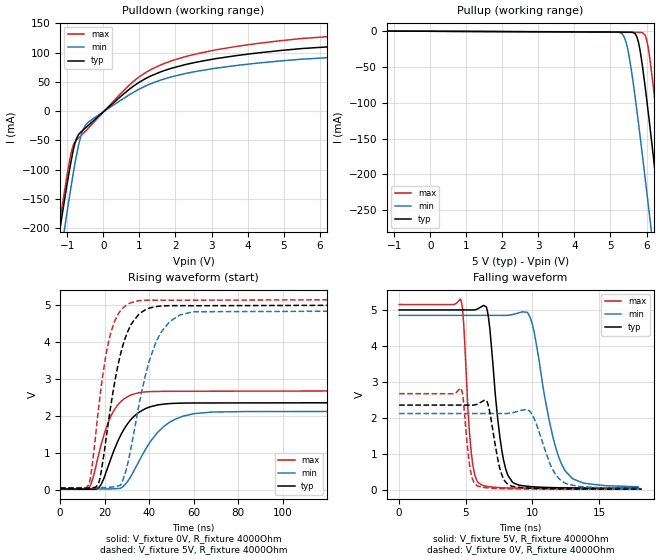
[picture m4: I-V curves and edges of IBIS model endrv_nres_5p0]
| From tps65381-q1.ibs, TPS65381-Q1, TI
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|   endrv_nres_5p0 Model
[Model]   endrv_nres_5p0
Model_type   Output
Polarity   Non-Inverting
Vmeas = 1.65
Vref = 2.5
Cref = 2pF
Rref = 50
|   typ   min   max
|   (nom PVT)   (fast PVT)   (slow PVT)
C_comp   1.702e-12   1.384e-12   1.872e-12
| Where nom  PVT is Nominal Process, 5V, 27C
|   Fast PVT is Strong Process,  5.15V, -40C
|   Slow PVT is Weak Process,   4.85V, 150C
[Voltage Range]   5   4.85   5.15
|Junction Temperature
[Temperature Range]   27   150   -40
[Pullup Reference]   5   4.85   5.15
[Pulldown Reference]   0   0   0
[Power Clamp Reference]   5   4.85   5.15
[GND Clamp Reference]   0   0   0
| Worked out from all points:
|   slope of the pulldown table from 0 to 0.75 V, typ, clamps not added: 18.8 ohm
|   slope of the pullup table from 0 to 0.75 V, typ, clamps not added: 4.48 kohm
|   falling waveform, V_fixture 5V, R_fixture 4000Ohm: 20-80 % time 815ps typ, 1.5ns min, 492ps max; typ from 5 V to 0.053 V
|   rising waveform, V_fixture 0V, R_fixture 4000Ohm: 20-80 % time 11ns typ, 14ns min, 8.45ns max; typ from 0.02 V to 2.36 V
|   rising waveform, V_fixture 5V, R_fixture 4000Ohm: 20-80 % time 8.92ns typ, 11ns min, 7.09ns max; typ from 0.043 V to 5 V
|   falling waveform, V_fixture 0V, R_fixture 4000Ohm: 20-80 % time 714ps typ, 1.29ns min, 445ps max; typ from 2.36 V to 0.025 V
[Pulldown]
|   Voltage   I(typ)   I(min)   I(max)
-5V       -1.931A    -1.927A    -1.96A
-1.232V   -211.8mA   -265.5mA   -197mA
-1.06V    -144.2mA   -193.9mA   -129.2mA
-882.3mV  -80.85mA   -123.2mA   -67.84mA
-760mV    -48.91mA   -79.67mA   -50.34mA
-625.3mV  -35.56mA   -42.43mA   -42.13mA
-500mV    -28.71mA   -24.43mA   -34.3mA
809.2mV   41.63mA    31.33mA    49.58mA
1.698V    69.52mA    55.27mA    81.68mA
2.617V    84.16mA    68.42mA    98.35mA
4.291V    99.53mA    82.16mA    115.8mA
10V       124.5mA    104.8mA    143.4mA
[Pullup]
|   Voltage   I(typ)   I(min)   I(max)
-5V       1.116mA    973.5uA    1.352mA
5.263V    -1.174mA   -1.864mA   -1.423mA
5.389V    -1.203mA   -9.349mA   -1.457mA
5.506V    -1.236mA   -32.1mA    -1.489mA
5.73V     -7.607mA   -109.9mA   -1.552mA
5.89V     -50.12mA   -175.1mA   -2.045mA
6.006V    -95.75mA   -224mA     -12.31mA
6.098V    -135.2mA   -263.8mA   -40.86mA
6.38V     -260.6mA   -385.9mA   -163.4mA
6.546V    -335.9mA   -458.5mA   -240.9mA
7.36V     -705.8mA   -815.7mA   -623.3mA
10V       -1.928A    -1.994A    -1.885A
[Ramp]
R_load = 4000
|   typ   min   max
dV/dt_r   1.40274/1.1037e-08   1.26021/1.39513e-08   1.59289/8.45493e-09
dV/dt_f   2.97234/8.11143e-10   2.87447/1.5107e-09   3.06466/4.90925e-10
[Falling Waveform]
V_fixture = 5V
V_fixture_min = 4.85V
V_fixture_max = 5.15V
R_fixture = 4000Ohm
|   Time   V(typ)   V(min)   V(max)
0s        5V         4.85V      5.15V
4.625ns   5V         4.85V      5.283V
5.35ns    4.999V     4.85V      1.287V
5.9ns     5.031V     4.85V      219mV
6.625ns   4.966V     4.85V      100mV
7.7ns     1.112V     4.849V     63.78mV
8.5ns     220.9mV    4.871V     55.01mV
9.975ns   92.02mV    4.636V     48.67mV
12.47ns   60.8mV     523.3mV    45.89mV
17.93ns   52.69mV    89.47mV    45.01mV
[Rising Waveform]
V_fixture = 0V
V_fixture_min = 0V
V_fixture_max = 0V
R_fixture = 4000Ohm
|   Time   V(typ)   V(min)   V(max)
0s        20.13mV    22.93mV    20.97mV
13ns      13.81mV    16.38mV    50.63mV
17.37ns   56.21mV    17.44mV    963.2mV
21.07ns   545.8mV    19.36mV    1.731V
24.3ns    1.077V     24.37mV    2.152V
29.43ns   1.703V     154.6mV    2.48V
35.37ns   2.089V     761.7mV    2.618V
46.78ns   2.312V     1.716V     2.656V
60.25ns   2.342V     2.055V     2.659V
249.3ns   2.356V     2.119V     2.674V
[Rising Waveform]
V_fixture = 5V
V_fixture_min = 4.85V
V_fixture_max = 5.15V
R_fixture = 4000Ohm
|   Time   V(typ)   V(min)   V(max)
0s        42.68mV    52.37mV    40.36mV
12.98ns   43.21mV    48.89mV    148mV
17.33ns   180.9mV    52.92mV    2.219V
20.63ns   1.367V     58.9mV     3.647V
23.82ns   2.665V     72.74mV    4.443V
27.9ns    3.834V     212.7mV    4.89V
32.08ns   4.482V     1.191V     5.057V
42.65ns   4.941V     3.921V     5.119V
53.77ns   4.973V     4.719V     5.118V
241.9ns   4.998V     4.846V     5.15V
[Falling Waveform]
V_fixture = 0V
V_fixture_min = 0V
V_fixture_max = 0V
R_fixture = 4000Ohm
|   Time   V(typ)   V(min)   V(max)
0s        2.358V     2.123V     2.676V
4.625ns   2.358V     2.123V     2.821V
5.35ns    2.357V     2.123V     548.7mV
5.9ns     2.389V     2.123V     108.8mV
6.6ns     2.452V     2.123V     60.53mV
7.6ns     541.3mV    2.123V     38.28mV
8.425ns   109.2mV    2.138V     31.48mV
9.85ns    51.23mV    2.168V     26.63mV
12.37ns   30.86mV    207mV      24.25mV
18.2ns    25.06mV    40.56mV    23.47mV
